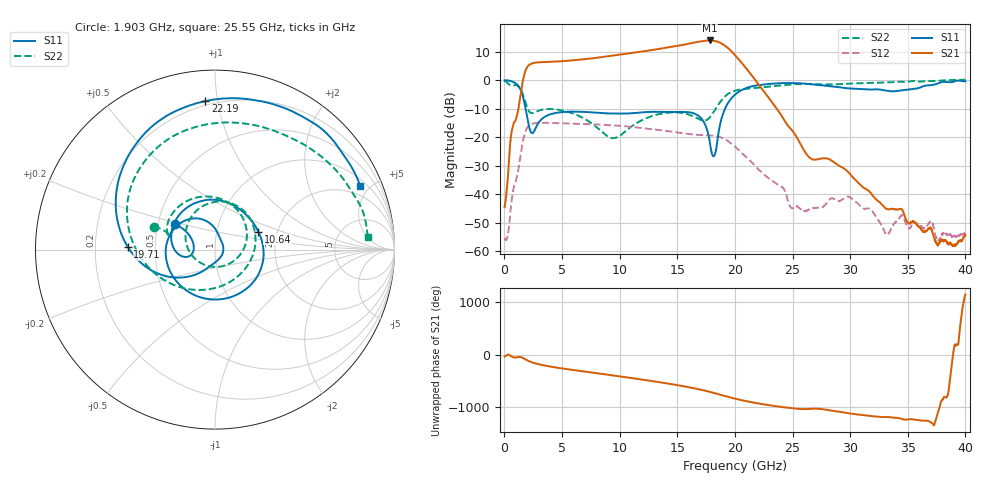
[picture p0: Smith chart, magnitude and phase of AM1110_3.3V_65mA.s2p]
!Agilent Technologies,E8364B,MY43040894,A.07.50.67
!Agilent E8364B: A.07.50.67
!Date: Wednesday, December 30, 2020 12:23:11
!Correction: S11(Full 2 Port(1,2))
!S21(Full 2 Port(1,2))
!S12(Full 2 Port(1,2))
!S22(Full 2 Port(1,2))
!S2P File: Measurements: S11, S21, S12, S22:
# Hz S  dB  R 50
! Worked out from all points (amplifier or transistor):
!   6401 points, 10 MHz to 40 GHz, reference 50 ohm
!   highest |S21| = 13.9 dB at 17.8 GHz (marker M1)
!   |S21| within 3 dB of that: 13.37 GHz to 19.49 GHz (6.12 GHz wide, 37.3 % of centre)
!   unconditionally stable (mu >= 1): start of sweep to 38.2 GHz
!   at 6.671 GHz: K = 1.35, MAG = 7.7 dB, |S12| = -15.3 dB
!   at 20 GHz: K = 1.34, MAG = 12.6 dB, |S12| = -23.3 dB
!   at 40 GHz: K = -418.72, MSG = -0.2 dB, |S12| = -53.8 dB
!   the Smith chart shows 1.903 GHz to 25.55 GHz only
!   S11 on the Smith chart (normalised r, x): 1.903 GHz: 0.61, +0.19; 10.64 GHz: 1.59, +0.34; 19.71 GHz: 0.35, +0.01; 22.19 GHz: 0.17, +0.92; 25.55 GHz: 1.34, +4.38
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1e7  -0.04 -9.8  -44.49 -38.8  -55.28 -52.0  -0.21 -13.1
7.723094e8  -0.64 -90.3  -15.31 -50.8  -38.02 169.2  -1.84 -91.8
1.903277e9  -11.55 147.6  4.10 -100.0  -17.12 95.6  -8.77 159.8
3.215448e9  -13.68 -173.4  6.32 164.6  -14.91 -5.5  -10.35 149.3
4.852539e9  -11.22 141.3  6.63 102.2  -15.03 -71.2  -10.46 99.4
6.677083e9  -11.05 98.7  7.24 46.1  -15.28 -128.7  -12.94 43.1
8.732819e9  -11.58 59.0  8.23 -14.5  -15.64 171.4  -19.02 -44.0
1.064484e10  -11.66 22.7  9.33 -72.5  -16.18 116.4  -17.37 -168.8
1.201325e10  -11.24 -11.3  10.10 -115.9  -16.80 77.5  -13.84 140.2
1.334417e10  -11.08 -57.5  10.92 -160.1  -17.41 39.8  -11.93 104.3
1.48063e10  -11.12 -121.2  11.87 147.8  -18.16 -2.4  -11.27 67.6
1.62122e10  -11.35 171.6  12.99 92.2  -18.93 -43.9  -12.37 22.0
1.701825e10  -13.11 129.4  13.61 55.3  -19.19 -69.0  -13.87 -24.3
1.77993e10  -21.16 78.0  13.93 14.5  -19.33 -96.9  -13.10 -96.7
1.884279e10  -13.36 -135.2  12.86 -48.0  -20.11 -142.3  -6.99 178.0
1.970508e10  -6.27 178.3  10.08 -99.1  -22.28 176.8  -4.12 131.0
2.0005e10  -5.06 165.0  8.81 -115.5  -23.27 163.6  -3.67 118.4
2.219195e10  -1.63 93.8  -2.20 147.4  -31.80 78.3  -2.59 61.5
2.554736e10  -1.07 23.6  -21.29 50.1  -44.67 26.3  -1.37 4.9
2.667208e10  -1.40 3.5  -27.64 52.5  -44.89 5.9  -1.34 -13.3
3.333917e10  -3.77 -102.5  -45.27 -105.2  -53.49 -127.5  -0.75 -113.5
4e10  -0.38 169.9  -54.24 59.0  -53.85 55.8  0.17 173.1
